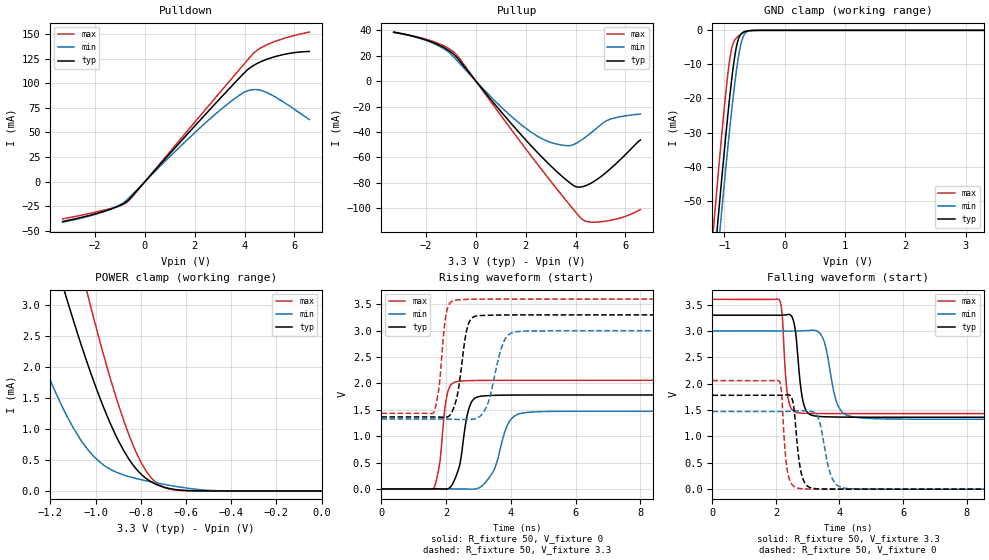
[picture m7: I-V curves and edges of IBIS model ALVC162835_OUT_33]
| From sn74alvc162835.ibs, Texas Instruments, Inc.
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[Model]   ALVC162835_OUT_33
Model_type  3-state
Enable   Active-Low
Vref =   0
Rref =   500
Cref =   50p
Vmeas =   1.5
| variable   typ   min   max
C_comp   5.72pF   4.72pF   7.31pF
| C_pullup   4.44pF   3.26pF   6.90pF
| C_pulldown   3.92pF   3.04pF   5.44pF
| C_tri-state   5.72pF   4.72pF   7.31pF
[Temperature Range]   40   100   -40
| Ambient temperature   25   85   -40
[Voltage range]   3.3   3   3.6
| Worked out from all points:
|   slope of the pulldown table from 0 to 0.495 V, typ, clamps not added: 35.1 ohm
|   slope of the pullup table from 0 to 0.495 V, typ, clamps not added: 41.5 ohm
|   GND clamp passes 1 mA (typ) near -0.72 V on its own axis
|   POWER clamp passes 1 mA (typ) near -0.92 V on its own axis
|   rising waveform, R_fixture 50, V_fixture 0: 20-80 % time 289ps typ, 451ps min, 209ps max; typ from 0 V to 1.78 V
|   falling waveform, R_fixture 50, V_fixture 3.3: 20-80 % time 193ps typ, 328ps min, 136ps max; typ from 3.3 V to 1.36 V
|   rising waveform, R_fixture 50, V_fixture 3.3: 20-80 % time 266ps typ, 392ps min, 195ps max; typ from 1.36 V to 3.3 V
|   falling waveform, R_fixture 50, V_fixture 0: 20-80 % time 192ps typ, 298ps min, 146ps max; typ from 1.78 V to 0 V
[GND Clamp]
| ALVC162835_OUT_33
|   Voltage   I(typ)   I(min)   I(max)
-3.3V     -530.6mA   -531.8mA   -526mA
-1.185V   -71.45mA   -80.34mA   -58.91mA
-1.165V   -67.4mA    -76.38mA   -54.77mA
-1.125V   -59.36mA   -68.51mA   -46.59mA
-1.105V   -55.38mA   -64.61mA   -42.55mA
-1.07V    -48.5mA    -57.85mA   -35.6mA
-965mV    -28.72mA   -38.25mA   -16.28mA
-890mV    -16.04mA   -25.23mA   -6.187mA
-790mV    -3.959mA   -10.43mA   -2.053mA
-680mV    -483.7uA   -1.522mA   -661.2uA
-490mV    -14.28uA   -17.14uA   -30.62uA
3.3V      818.4pA    26.03nA    9.52nA
[POWER Clamp]
| ALVC162835_OUT_33
|   Voltage   I(typ)   I(min)   I(max)
-3.3V     42.81mA    34.14mA    51.3mA
-1.355V   6.151mA    3.289mA    8.476mA
-1.33V    5.791mA    3.026mA    8.024mA
-1.125V   3.076mA    1.199mA    4.543mA
-1.04V    2.104mA    695.6uA    3.248mA
-1.03V    1.998mA    649.8uA    3.103mA
-935mV    1.093mA    351uA      1.823mA
-855mV    529.3uA    234uA      932.5uA
-795mV    258.9uA    178.5uA    437.1uA
-735mV    110.6uA    132.9uA    143.8uA
-625mV    13.01uA    61.53uA    7.719uA
-48.03fV  818.4pA    33.32pA    9.031nA
[Pulldown]
| ALVC162835_OUT_33
|   Voltage   I(typ)   I(min)   I(max)
-3.3V     -40.43mA   -41.1mA    -37.73mA
-1.595V   -29.7mA    -29.87mA   -28.59mA
-1.015V   -24.37mA   -23.63mA   -24.45mA
-680mV    -19.05mA   -17.46mA   -19.95mA
1.03V     29.29mA    26.17mA    31.17mA
2.295V    64.66mA    56.58mA    69.22mA
3.4V      94.85mA    80.5mA     102.2mA
4.065V    112.4mA    91.76mA    122mA
4.435V    119.1mA    93.53mA    132.1mA
4.875V    124.1mA    90.81mA    138.8mA
5.71V     129.9mA    78.5mA     146.5mA
6.6V      132.3mA    63.12mA    152mA
[Pullup]
| ALVC162835_OUT_33
|   Voltage   I(typ)   I(min)   I(max)
-3.3V     38.48mA    38.53mA    38.18mA
-1.735V   30.49mA    29.91mA    31.27mA
-815mV    19.64mA    17.37mA    21.57mA
900mV     -21.47mA   -18.14mA   -24.23mA
2.155V    -49.5mA    -39.24mA   -57.15mA
3.105V    -68.49mA   -48.8mA    -81.19mA
3.68V     -78.49mA   -50.74mA   -95.26mA
3.985V    -82.7mA    -49.24mA   -102.5mA
4.34V     -82.62mA   -44.84mA   -109.5mA
4.79V     -78.19mA   -37.92mA   -110.8mA
5.39V     -68.99mA   -29.92mA   -109.4mA
6.6V      -46.27mA   -25.85mA   -100.9mA
[Ramp]
| ALVC162835_OUT_33
| variable   typ   min   max
dV/dt_r   1.07/2.98E-10   0.89/4.58E-10   1.24/2.12E-10
dV/dt_f   1.17/1.99E-10   1.01/3.36E-10   1.30/1.38E-10
R_load = 50
[Rising Waveform]
| ALVC162835_OUT_33
R_fixture =   50
C_fixture =   0
L_fixture =   0
V_fixture =   0
V_fixture_min = 0
V_fixture_max = 0
|   Time   V(typ)   V(min)   V(max)
0s        17.49pV    37.88pV    15.12pV
1.62ns    685.9uV    -42.05uV   17.8mV
1.815ns   -19.54uV   217.9uV    542.4mV
2.03ns    -1.401mV   1.593mV    1.783V
2.36ns    330.1mV    -386.8uV   2.038V
2.705ns   1.525V     -3.97mV    2.053V
3.095ns   1.76V      50.51mV    2.057V
3.935ns   1.779V     1.259V     2.059V
4.43ns    1.78V      1.446V     2.059V
20ns      1.781V     1.473V     2.059V
[Falling Waveform]
| ALVC162835_OUT_33
R_fixture =   50
C_fixture =   0
L_fixture =   0
V_fixture =   3.3
V_fixture_min = 3
V_fixture_max = 3.6
|   Time   V(typ)   V(min)   V(max)
0s        3.3V       3V         3.6V
2.11ns    3.298V     3V         3.59V
2.2ns     3.3V       2.999V     3.286V
2.375ns   3.312V     2.998V     1.754V
2.685ns   2.547V     3V         1.45V
2.995ns   1.454V     3.008V     1.437V
3.45ns    1.376V     2.897V     1.435V
3.94ns    1.368V     1.604V     1.434V
4.455ns   1.366V     1.367V     1.434V
20ns      1.365V     1.326V     1.433V
[Rising Waveform]
| ALVC162835_OUT_33
R_fixture =   50
C_fixture =   0
L_fixture =   0
V_fixture =   3.3
V_fixture_min = 3
V_fixture_max = 3.6
|   Time   V(typ)   V(min)   V(max)
0s        1.365V     1.326V     1.433V
1.62ns    1.365V     1.326V     1.453V
1.775ns   1.363V     1.326V     1.894V
2ns       1.358V     1.325V     3.309V
2.27ns    1.598V     1.32V      3.577V
2.64ns    3.017V     1.317V     3.594V
2.935ns   3.279V     1.335V     3.597V
3.78ns    3.298V     2.792V     3.6V
4.135ns   3.299V     2.977V     3.6V
20ns      3.3V       3V         3.6V
[Falling Waveform]
| ALVC162835_OUT_33
R_fixture =   50
C_fixture =   0
L_fixture =   0
V_fixture =   0
V_fixture_min = 0
V_fixture_max = 0
|   Time   V(typ)   V(min)   V(max)
0s        1.781V     1.473V     2.059V
2.11ns    1.781V     1.473V     2.046V
2.37ns    1.79V      1.474V     318.4mV
2.545ns   1.624V     1.48V      63.13mV
2.735ns   514.5mV    1.486V     14.34mV
2.91ns    118.5mV    1.486V     4.613mV
3.305ns   7.414mV    1.389V     926uV
3.74ns    1.693mV    246.5mV    302.5uV
4.175ns   556uV      17.28mV    97.88uV
20ns      1.221nV    -5.998nV   -1.359nV
